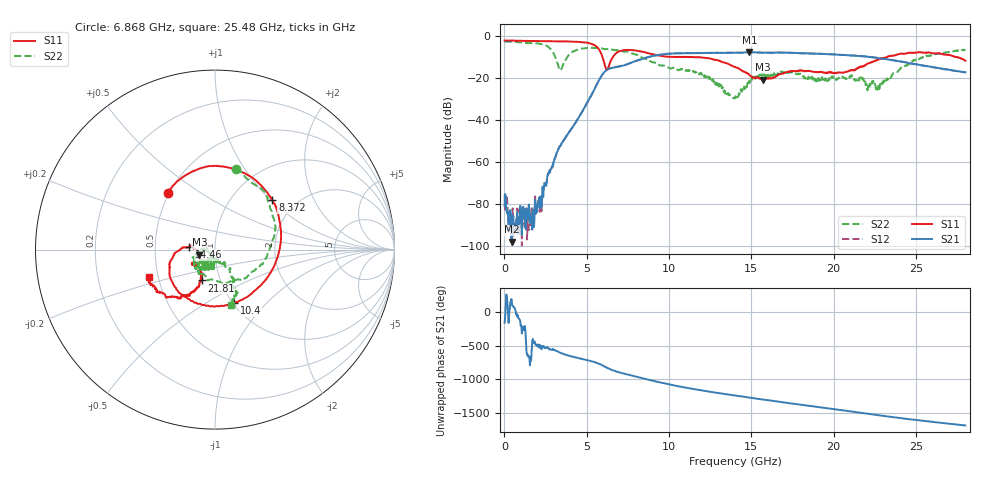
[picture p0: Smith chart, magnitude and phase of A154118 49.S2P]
!  2-Port S-parameters saved by WinCal
! VAR MeasName=S-Parameters (CALIBRATED_DATA) read from VNA (N5230A)
! VAR MeasDate=2015-9-10 14:38:20
! VAR NAME=A154118 49
! VAR FILENAME=A154118 49.S2P
! VAR DATE=2015-9-10 14:38:20
! VAR PHYS_PORTS=1,2
# Hz S DB R 50
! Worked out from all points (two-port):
!   801 points, 10 MHz to 28 GHz, reference 50 ohm
!   highest |S21| = -7.76 dB at 14.88 GHz (marker M1); lowest = -98.1 dB at 429.9 MHz (marker M2)
!   |S21| within 3 dB of the highest: 8.438 GHz to 22.91 GHz (14.47 GHz wide, 92.3 % of centre)
!   lowest |S11| = -20.8 dB at 15.72 GHz (marker M3), VSWR 1.20, Z = 41.9 - j2.38 ohm
!   |S11| at or under -10 dB: 5.957 GHz to 6.588 GHz (630.4 MHz wide, 10.1 % of centre); 11.34 GHz to 23.26 GHz (11.92 GHz wide, 68.9 % of centre); 27.48 GHz to end of sweep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
!   |S22| runs from -30.0 to -2.7 dB; largest |S21 - S12| = 0.0088
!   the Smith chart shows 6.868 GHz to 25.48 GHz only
!   S11 on the Smith chart (normalised r, x): 6.868 GHz: 0.49, +0.38; 8.372 GHz: 1.53, +1.02; 10.4 GHz: 1.01, -0.67; 14.46 GHz: 0.75, +0.02; 21.81 GHz: 0.82, -0.29; 25.48 GHz: 0.44, -0.16
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1e7  -2.15 179.7  -81.01 -156.1  -75.95 115.8  -2.67 179.8
4.2985e8  -2.22 173.8  -98.09 -160.5  -84.84 49.5  -2.75 169.5
2.144238e9  -2.45 151.6  -82.09 -124.7  -83.84 178.3  -3.68 122.1
3.0889e9  -2.51 136.6  -57.79 149.6  -57.78 149.7  -10.05 37.2
3.613712e9  -2.62 126.6  -49.52 94.7  -49.43 95.3  -12.80 -119.2
4.698325e9  -3.00 98.3  -36.43 25.1  -36.42 25.2  -5.98 154.0
5.74795e9  -6.49 27.3  -21.06 -50.4  -21.03 -50.2  -5.69 115.2
6.237775e9  -16.11 -109.4  -16.10 -110.5  -16.01 -110.5  -6.24 98.4
6.86755e9  -7.73 129.5  -14.72 -171.1  -14.67 -171.5  -6.71 75.4
8.372012e9  -7.51 40.7  -10.92 94.6  -10.94 94.3  -10.34 0.4
9.351662e9  -9.29 -14.0  -9.09 37.0  -9.05 36.7  -13.71 -53.7
1.040129e10  -10.05 -70.4  -8.30 -19.0  -8.27 -19.3  -15.47 -104.7
1.211568e10  -10.38 -140.1  -8.11 -93.9  -8.06 -94.6  -19.38 -162.7
1.4005e10  -14.76 176.5  -8.00 -164.9  -7.98 -165.5  -29.36 -132.8
1.445984e10  -16.87 174.3  -7.95 179.7  -7.96 178.9  -24.73 -99.2
1.487969e10  -18.59 176.9  -7.76 164.0  -7.74 163.2  -21.31 -92.9
1.571939e10  -20.77 -162.1  -7.96 134.4  -7.97 133.8  -19.13 -105.1
1.869332e10  -16.90 -146.5  -8.38 34.5  -8.40 34.1  -19.54 -128.9
2.180721e10  -14.56 -113.4  -9.67 -68.6  -9.68 -69.3  -20.26 -112.2
2.334666e10  -9.73 -125.0  -11.26 -120.5  -11.16 -121.8  -20.48 -51.1
2.54809e10  -7.98 -157.1  -14.16 175.5  -14.18 174.0  -9.85 -74.1
2.8e10  -11.81 164.3  -17.28 106.9  -17.37 105.8  -6.39 -102.8
